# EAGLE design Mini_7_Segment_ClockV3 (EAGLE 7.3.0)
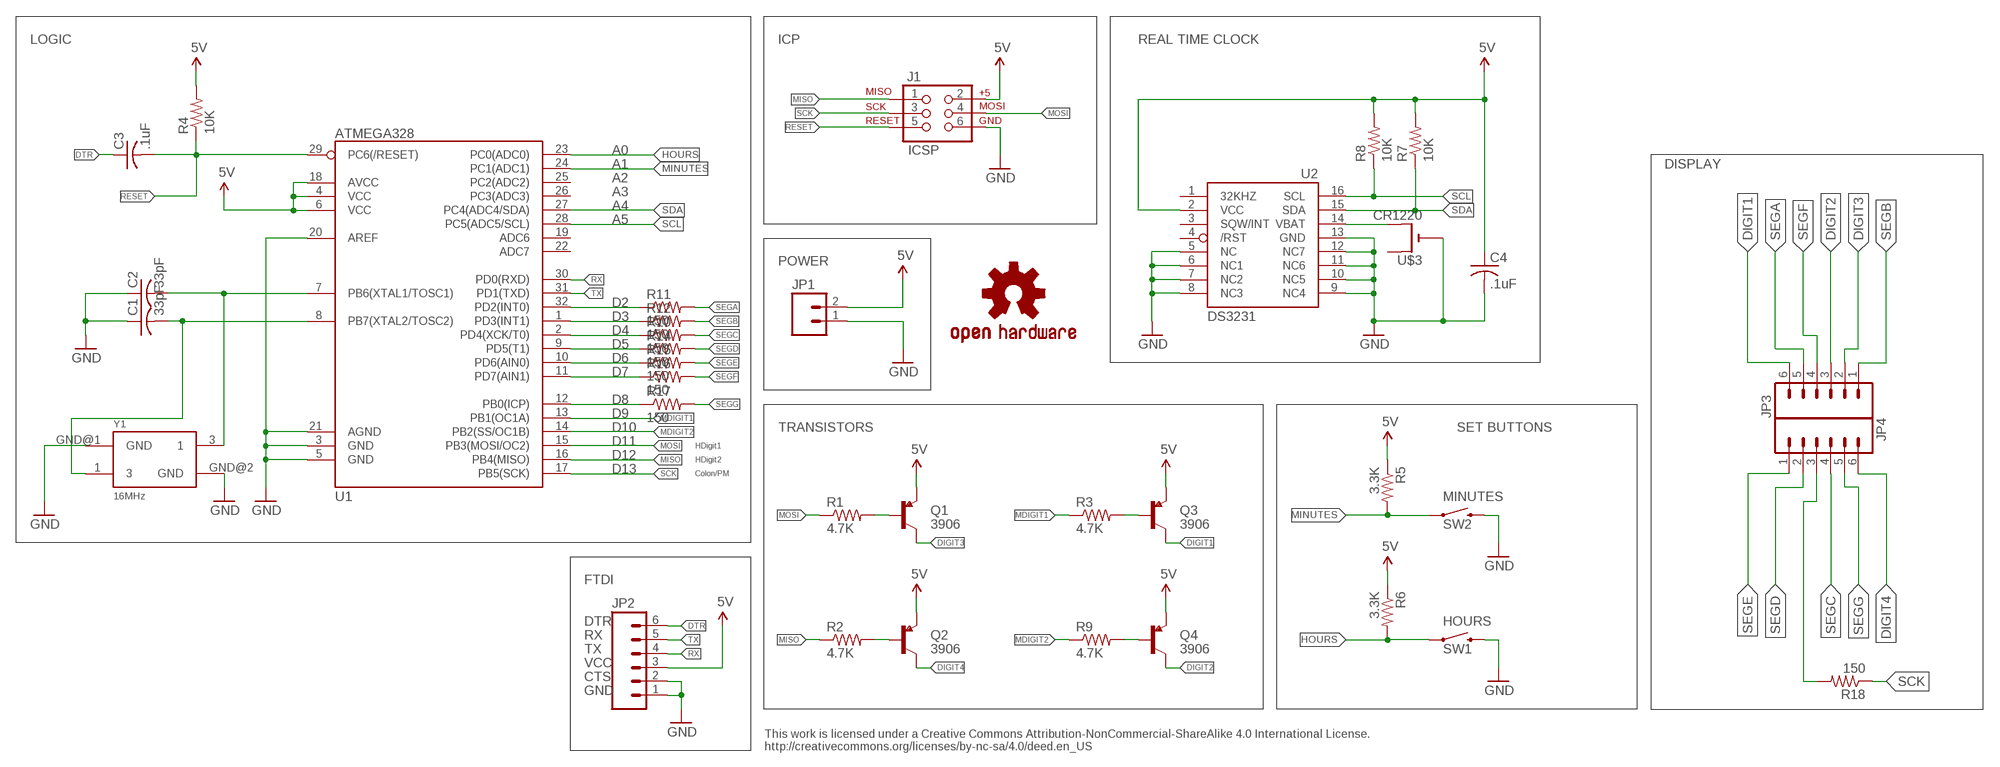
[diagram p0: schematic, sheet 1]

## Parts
C1  33pF  C-USC0805K  [C0805K]
C2  33pF  C-USC0805K  [C0805K]
C3  .1uF  C-USC0805K  [C0805K]
C4  .1uF  C-USC0805K  [C0805K]
HOURS  SW1  SWITCH-MOMENTARY-2PTH  [TACTILE-PTH]
J1  ICSP  AVR_SPI_PRG_6PTH  [2X3]
JP1  M02PTH  [1X02]
JP2  M06NO_SILK_FEMALE_PTH  [1X06_NO_SILK]
JP3  M06NO_SILK_FEMALE_PTH  [1X06_NO_SILK]
JP4  M06NO_SILK_FEMALE_PTH  [1X06_NO_SILK]
MINUTES  SW2  SWITCH-MOMENTARY-2PTH  [TACTILE-PTH]
Q1  3906  TRANSISTOR_PNPPMBT3906  [SOT23-3]
Q2  3906  TRANSISTOR_PNPPMBT3906  [SOT23-3]
Q3  3906  TRANSISTOR_PNPPMBT3906  [SOT23-3]
Q4  3906  TRANSISTOR_PNPPMBT3906  [SOT23-3]
R1  4.7K  R-US_R0805  [R0805]
R2  4.7K  R-US_R0805  [R0805]
R3  4.7K  R-US_R0805  [R0805]
R4  10K  R-US_R0805  [R0805]
R5  3.3K  R-US_R0805  [R0805]
R6  3.3K  R-US_R0805  [R0805]
R7  10K  R-US_R0805  [R0805]
R8  10K  R-US_R0805  [R0805]
R9  4.7K  R-US_R0805  [R0805]
R10  150  R-US_R0805  [R0805]
R11  150  R-US_R0805  [R0805]
R12  150  R-US_R0805  [R0805]
R14  150  R-US_R0805  [R0805]
R15  150  R-US_R0805  [R0805]
R16  150  R-US_R0805  [R0805]
R17  150  R-US_R0805  [R0805]
R18  150  R-US_R0805  [R0805]
U1  ATMEGA328  ATMEGA328_SMT  [TQFP32-08]
U2  DS3231  DS3231/SO  [SO16W]
U$3  CR1220  CR1220SMT  [CR1220-SMD]
U$7  OSHW-LOGOS  [OSHW-LOGO-S]
Y1  16MHz  OSCILLATOR5X3  [CRYSTAL-SMD-5X3]

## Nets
5V: C4.1 J1.2 JP1.2 JP2.3 Q1.2(E) Q2.2(E) Q3.2(E) Q4.2(E) R4.2 R5.1 R6.1 R7.2 R8.2 U1.4(VCC) U1.6(VCC) U1.18(AVCC) U2.2(VCC)
DIGIT1: JP3.6 Q3.3(C)
DIGIT2: JP3.3 Q4.3(C)
DIGIT3: JP3.2 Q1.3(C)
DIGIT4: JP4.6 Q2.3(C)
DTR: C3.1 JP2.6
GND: C1.1 C2.1 C4.2 HOURS.3 J1.6 JP1.1 JP2.1 JP2.2 MINUTES.3 U1.3(GND) U1.5(GND) U1.20(AREF) U1.21(AGND) U2.5(NC) U2.6(NC1) U2.7(NC2) U2.8(NC3) U2.9(NC4) U2.10(NC5) U2.11(NC6) U2.12(NC7) U2.13(GND) U$3.- Y1.GND@1(GND) Y1.GND@2(GND)
HOURS: HOURS.1 R6.2 U1.23(PC0(ADC0))
MDIGIT1: R3.1 U1.13(PB1(OC1A))
MDIGIT2: R9.1 U1.14(PB2(SS/OC1B))
MINUTES: MINUTES.1 R5.2 U1.24(PC1(ADC1))
MISO: J1.1 R2.1 U1.16(PB4(MISO))
MOSI: J1.4 R1.1 U1.15(PB3(MOSI/OC2))
N$1: R10.1 U1.2(PD4(XCK/T0))
N$2: JP4.3 R18.2
N$3: Q1.1(B) R1.2
N$4: R12.1 U1.1(PD3(INT1))
N$5: Q2.1(B) R2.2
N$6: Q3.1(B) R3.2
N$7: Q4.1(B) R9.2
N$8: C1.2 U1.8(PB7(XTAL2/TOSC2)) Y1.1
N$9: R16.1 U1.11(PD7(AIN1))
N$10: C2.2 U1.7(PB6(XTAL1/TOSC1)) Y1.3
N$11: R17.1 U1.12(PB0(ICP))
N$12: R14.1 U1.9(PD5(T1))
N$13: R11.1 U1.32(PD2(INT0))
N$14: R15.1 U1.10(PD6(AIN0))
N$15: U2.14(VBAT) U$3.+$2(+1)
RESET: C3.2 J1.5 R4.1 U1.29(PC6(/RESET))
RX: JP2.4 U1.30(PD0(RXD))
SCK: J1.3 R18.1 U1.17(PB5(SCK))
SCL: R8.1 U1.28(PC5(ADC5/SCL)) U2.16(SCL)
SDA: R7.1 U1.27(PC4(ADC4/SDA)) U2.15(SDA)
SEGA: JP3.5 R11.2
SEGB: JP3.1 R12.2
SEGC: JP4.4 R10.2
SEGD: JP4.2 R14.2
SEGE: JP4.1 R15.2
SEGF: JP3.4 R16.2
SEGG: JP4.5 R17.2
TX: JP2.5 U1.31(PD1(TXD))
Unconnected: U1.19(ADC6) U1.22(ADC7) U1.25(PC2(ADC2)) U1.26(PC3(ADC3)) U2.1(32KHZ) U2.3(SQW/INT) U2.4(/RST) U$3.+$1(+)

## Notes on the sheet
- LOGIC | ICP | REAL TIME CLOCK
- A0
- A1 | DISPLAY
- A2
- A3
- A4
- A5
- POWER
- D2
- D3
- D4
- D5
- D6
- D7
- D8
- D9
- D10 | TRANSISTORS | SET BUTTONS
- D11 | HDigit1
- D12 | HDigit2
- D13 | Colon/PM
- FTDI
- DTR
- RX
- TX
- VCC
- CTS
- GND
- This work is licensed under a Creative Commons Attribution-NonCommercial-ShareAlike 4.0 International License.
  http://creativecommons.org/licenses/by-nc-sa/4.0/deed.en_US

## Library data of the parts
C1-C4 = adafruit:C-US: CAPACITOR, American symbol
HOURS MINUTES = SparkFun:SWITCH-MOMENTARY-2
J1 = SparkFun:AVR_SPI_PRG_6: AVR ISP 6 Pin This is the reduced ISP connector for AVR programming. Common on Arduino. This footprint will take up less PCB space and can be used with a 10-pin to 6-pin adapter such as SKU: BOB-08508; OC_NEWARK: unknown
JP1 = SparkFun-Connectors:M02: Header 2
JP2-JP4 = SparkFun-Connectors:M06: Header 6 Standard 6-pin 0.1" header. Use with straight break away headers (SKU : PRT-00116), right angle break away headers (PRT-00553), swiss pins (PRT-00743), machine pins (PRT-00117), and female headers (PRT-00115). Molex polarized connector foot print use with SKU : PRT-08094 with associated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; PROD_ID: CONN-08437
Q1-Q4 = SparkFun-DiscreteSemi:TRANSISTOR_PNP: Generic PNP BJT Double check pinouts against datasheets- not all devices are the same! MMBT3906 - 40V 200mA SOT-23 (TRANS-08052) MMBT4403 - 40V 600mA SOT-23 (TRANS-09245); PROD_ID: TRANS-08052; VALUE: PMBT3906
R1-R12 R14-R18 = adafruit:R-US_: RESISTOR, American symbol
U1 = SparkFun-DigitalIC:ATMEGA328_SMT: 32-Pin Atmega328 part Commonly used on Arduino compatible boards Available in QFP and QFN packages TQFP is IC-09069 QFN is non-stock; PROD_ID: IC-09069; VALUE: ATMEGA328P
U2 = adafruit:DS3231
U$3 = adafruit:CR1220: CR1216/CR1220/CR1225 12mm 3V lithium coin cell Great for battery packup. Both SMT and THM holders. Note the THM package has the ground pads on both sides of the PCB so that the masks are the same - this reduces the cost
U$7 = SparkFun:OSHW-LOGO: Open Source Hardware Logo This logo indicates the piece of hardware it is found on incorporates a OSHW license and/or adheres to the definition of open source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
Y1 = SparkFun-FreqCtrl:OSCILLATOR: Generic 5x3 and 7x5 oscillators

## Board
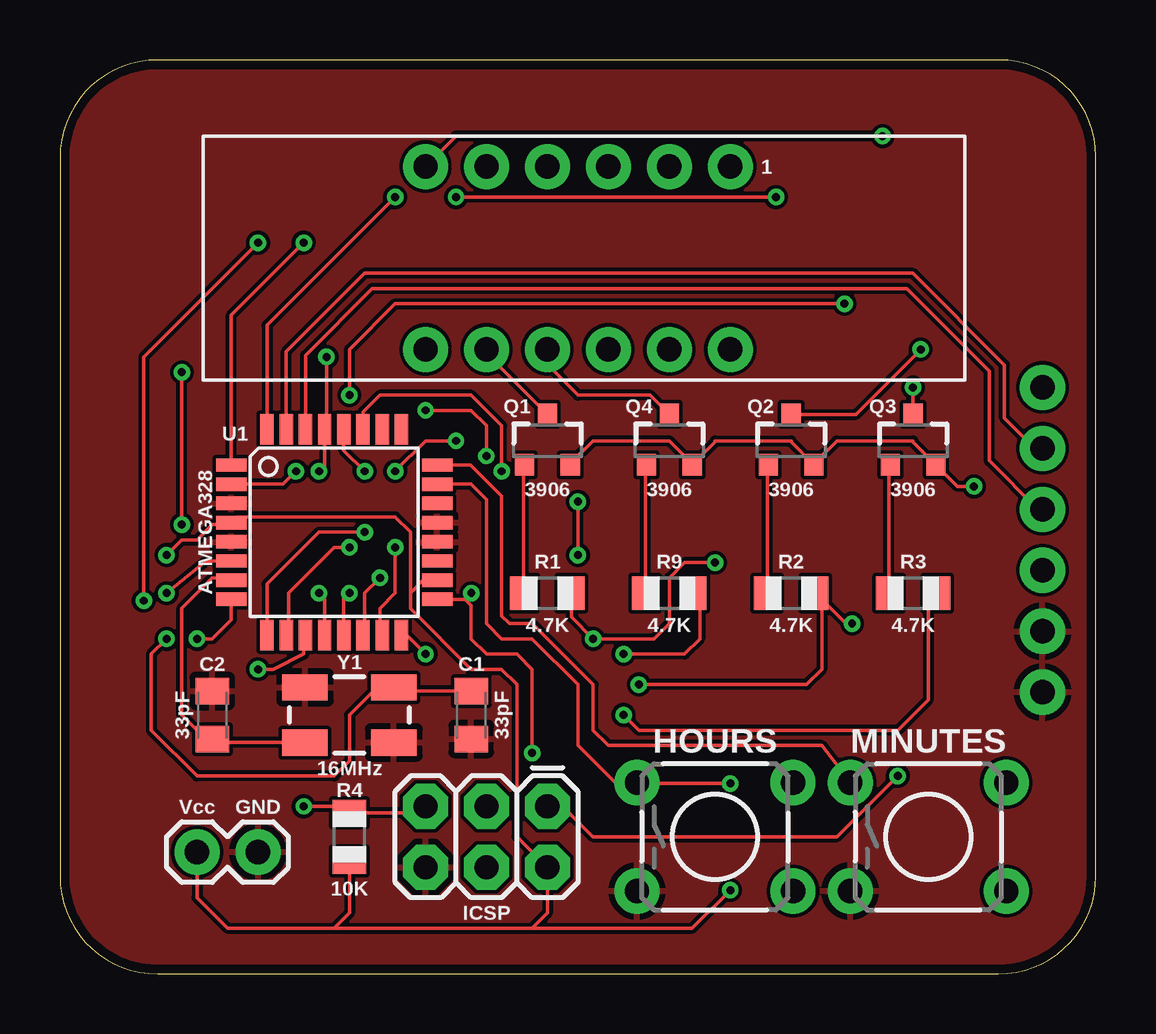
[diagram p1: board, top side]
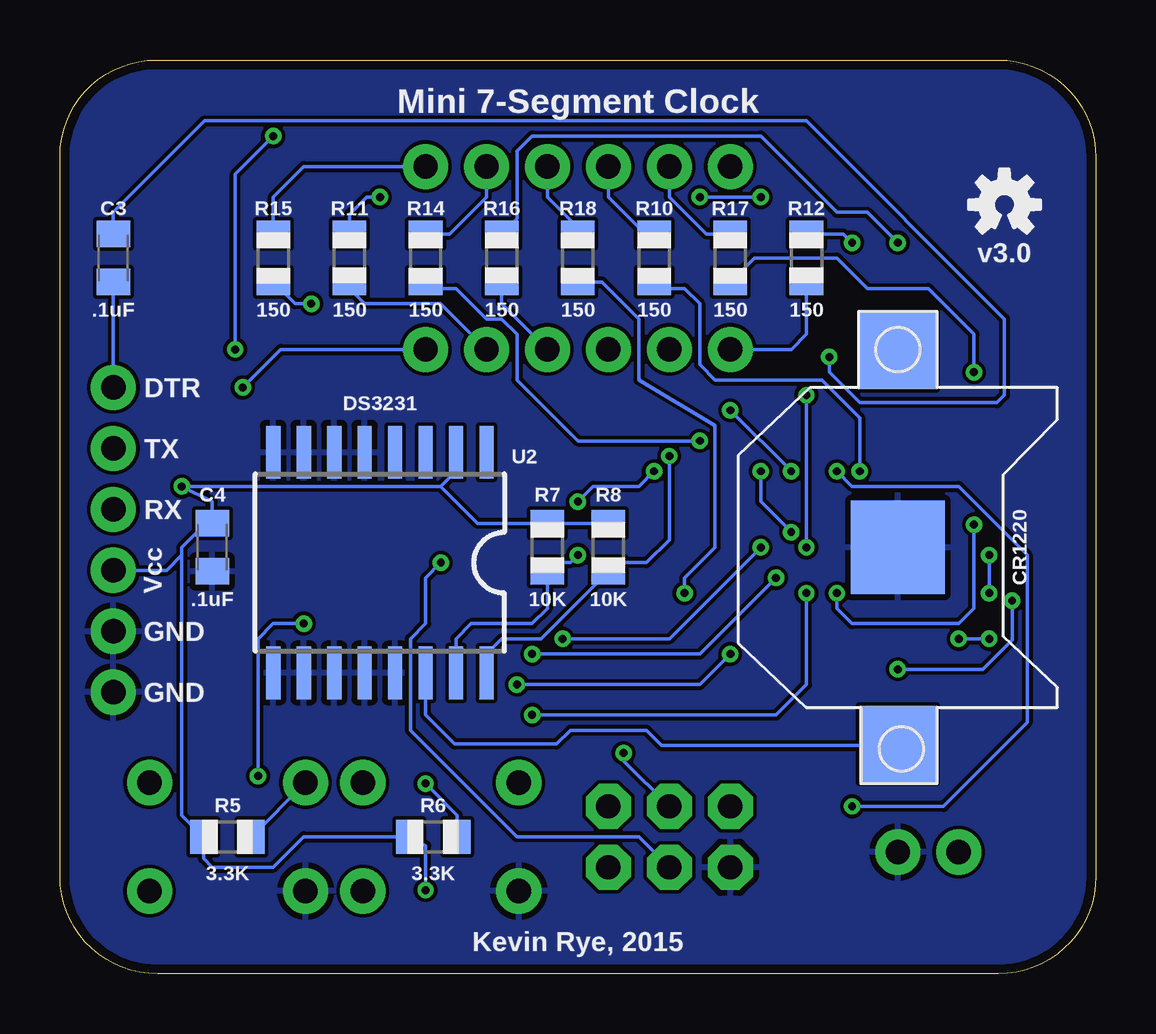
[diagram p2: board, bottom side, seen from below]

Size 43.18 x 38.1 mm. Coordinates in mm from the lower left corner, seen from the top.
Outline: 0,34.03 0,4.07 arc90 4.07,0 39.11,0 arc90 43.18,4.07 43.18,34.08 arc90 39.16,38.1 4.07,38.1 arc90 0,34.03
Copper layers (1*16): Top 0.0356mm / dielectric 1.5011mm / Bottom 0.0356mm
Design rules "LaenPCBOrder": minimum track width 6mil, minimum drill 13mil, track to track 6mil, track to pad 6mil, pad to pad 6mil, via to via 6mil, smd to smd 6mil, copper to edge 15mil, drill to drill 6mil, minimum pad ring 7mil, minimum via ring 7mil, stop-mask expansion 3mil, vias tented up to drill 0mil, thermal gap 10mil

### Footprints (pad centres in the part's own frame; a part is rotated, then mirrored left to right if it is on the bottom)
C0805K = smd 1.1 x 1.4: 1 -1,0; 2 1,0
TACTILE-PTH = drill 1.016 pad 1.88: 1 -3.251,2.261; 2 3.251,2.261; 3 -3.251,-2.261; 4 3.251,-2.261
2X3 = drill 1.016 pad 1.88 octagon: 1 0,0; 2 0,2.54; 3 2.54,0; 4 2.54,2.54; 5 5.08,0; 6 5.08,2.54
1X02 = drill 1.016 pad 1.88: 1 0,0; 2 2.54,0
1X06_NO_SILK = drill 1.016 pad 1.88: 1 0,0; 2 2.54,0; 3 5.08,0; 4 7.62,0; 5 10.16,0; 6 12.7,0
SOT23-3 = smd 0.8 x 0.9: 1 -0.95,-1; 2 0.95,-1; 3 0,1.1
R0805 = smd 1.1 x 1.4: 1 -1,0; 2 1,0
TQFP32-08 = smd 1.27 x 0.559: 1 -4.293,2.8; 2 -4.293,2; 3 -4.293,1.2; 4 -4.293,0.4; 5 -4.293,-0.4; 6 -4.293,-1.2; 7 -4.293,-2; 8 -4.293,-2.8; 17 4.293,-2.8; 18 4.293,-2; 19 4.293,-1.2; 20 4.293,-0.4; 21 4.293,0.4; 22 4.293,1.2; 23 4.293,2; 24 4.293,2.8 | smd 0.559 x 1.27: 9 -2.8,-4.293; 10 -2,-4.293; 11 -1.2,-4.293; 12 -0.4,-4.293; 13 0.4,-4.293; 14 1.2,-4.293; 15 2,-4.293; 16 2.8,-4.293; 25 2.8,4.293; 26 2,4.293; 27 1.2,4.293; 28 0.4,4.293; 29 -0.4,4.293; 30 -1.2,4.293; 31 -2,4.293; 32 -2.8,4.293
SO16W = smd 0.6 x 2.2: 1 -4.445,-4.6; 2 -3.175,-4.6; 3 -1.905,-4.6; 4 -0.635,-4.6; 5 0.635,-4.6; 6 1.905,-4.6; 7 3.175,-4.6; 8 4.445,-4.6; 9 4.445,4.6; 10 3.175,4.6; 11 1.905,4.6; 12 0.635,4.6; 13 -0.635,4.6; 14 -1.905,4.6; 15 -3.175,4.6; 16 -4.445,4.6
CR1220-SMD = smd 3.2 x 3.2: +$1 -8.2,0; +$2 8.2,0 | smd 3.9 x 3.9: - 0,0
CRYSTAL-SMD-5X3 = smd 1.9 x 1.1: 1 -1.85,-1.15; 3 1.85,1.15; GND@1 -1.85,1.15; GND@2 1.85,-1.15

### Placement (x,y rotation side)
C1  17.14,10.79 90 top
C2  6.35,10.79 270 top
C3  40.96,29.85 90 bottom
C4  36.83,17.78 270 bottom
HOURS  27.3,5.71 0 top
J1  20.32,6.98 180 top
JP1  8.26,5.08 180 top
JP2  40.96,11.75 90 bottom
JP3  15.24,26.04 0 top
JP4  27.94,33.66 180 top
MINUTES  36.2,5.71 0 top
Q1  20.32,22.23 0 top
Q2  30.48,22.23 0 top
Q3  35.56,22.23 0 top
Q4  25.4,22.23 0 top
R1  20.32,15.88 180 top
R2  30.48,15.88 180 top
R3  35.56,15.88 180 top
R4  12.06,5.71 270 top
R5  36.2,5.71 0 bottom
R6  27.62,5.71 0 bottom
R7  22.86,17.78 90 bottom
R8  20.32,17.78 90 bottom
R9  25.4,15.88 180 top
R10  18.41,29.85 90 bottom
R11  31.11,29.85 270 bottom
R12  12.06,29.85 270 bottom
R14  27.94,29.85 90 bottom
R15  34.29,29.85 90 bottom
R16  24.77,29.85 270 bottom
R17  15.24,29.85 90 bottom
R18  21.59,29.85 90 bottom
U1  11.43,18.42 0 top
U2  29.84,17.15 180 bottom
U$3  8.26,17.78 270 bottom
U$7  3.81,32.07 0 bottom
Y1  12.06,10.79 180 top

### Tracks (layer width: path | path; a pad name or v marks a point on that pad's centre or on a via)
5V  (via drill 0.33 pad 0.69)
  Top 0.152: JP1.2 5.71,3.17 6.98,1.91 11.43,1.91 | 11.43,1.91 19.68,1.91 | 19.68,1.91 26.35,1.91 v27.94,3.49 | 19.68,1.91 20.32,2.54 J1.2 19.05,5.71 19.05,12.06 18.41,12.7 17.14,12.7 14.61,15.24 14.61,15.88 | R4.2 12.06,2.54 11.43,1.91 | Q1.2 21.27,21.27 22.22,22.23 25.4,22.23 26.35,21.28 | 26.35,21.28 Q4.2 27.3,22.18 27.3,22.23 30.48,22.23 30.48,22.18 Q2.2 31.43,21.27 32.38,22.23 35.56,22.23 35.56,22.18 Q3.2 37.42,20.32 v38.1,20.32 | 26.35,21.28 26.36,21.28 | U1.6 6.1,17.21 v4.45,15.88 | U1.18 15.14,16.41 14.61,15.88 | 14.61,15.88 14.61,18.42 13.97,19.05 7.37,19.05 U1.4 7.05,18.73 6.35,18.73 5.71,18.1 5.08,18.1 v4.45,17.46
  Bottom 0.152: v27.94,3.49 27.94,5.35 R6.1 33.02,5.71 34.29,4.45 36.83,4.45 37.2,4.81 R5.1 38.1,6.62 38.1,17.46 | 38.1,17.46 38.1,17.78 37.1,18.78 C4.1 36.83,19.69 v38.1,20.32 27.3,20.32 | U2.2 26.67,20.96 27.3,20.32 | 27.3,20.32 25.77,18.78 R7.2 R8.2 | v4.45,15.88 v4.45,17.46 | JP2.3 38.74,16.83 38.1,17.46
DIGIT1  (via drill 0.33 pad 0.69)
  Top 0.152: Q3.3 v35.56,24.45
  Bottom 0.152: v35.56,24.45 33.97,26.04 JP3.6
DIGIT2
  Top 0.152: Q4.3 24.59,24.13 21.59,24.13 20.32,25.4 JP3.3
DIGIT3
  Top 0.152: Q1.3 17.78,25.87 JP3.2
DIGIT4  (via drill 0.33 pad 0.69)
  Top 0.152: Q2.3 33.17,23.33 v35.88,26.04 | v34.29,34.92 16.51,34.92 JP4.6
  Bottom 0.152: v35.88,26.04 35.88,33.34 v34.29,34.92
DTR
  Bottom 0.152: C3.1 JP2.6
GND
  pour Bottom: -0.64,38.73 43.82,39.05 43.82,-0.64 -0.64,-0.64
  pour Top: -0.32,38.42 43.5,38.42 43.5,-0.32 -0.32,-0.32
HOURS  (via drill 0.33 pad 0.69)
  Top 0.152: U1.23 17.14,20.42 17.78,19.77 17.78,14.61 18.41,13.97 19.68,13.97 21.59,12.06 21.59,9.53 23.14,7.98 HOURS.1 24.09,7.94 v27.94,7.94
  Bottom 0.152: R6.2 26.62,6.62 v27.94,7.94
MDIGIT1  (via drill 0.33 pad 0.69)
  Top 0.152: R3.1 36.2,15.88 36.2,11.43 34.93,10.16 24.13,10.16 v23.5,10.79 | v12.06,15.88 11.83,15.64 U1.13
  Bottom 0.152: v23.5,10.79 13.33,10.79 12.06,12.06 v12.06,15.88
MDIGIT2  (via drill 0.33 pad 0.69)
  Top 0.152: R9.1 26.67,15.61 26.67,13.97 26.04,13.33 v23.5,13.33 | v13.33,16.51 12.7,15.88 12.7,14.12 U1.14
  Bottom 0.152: v23.5,13.33 16.51,13.33 v13.33,16.51
MINUTES
  Top 0.152: U1.24 17.12,21.21 18.41,19.92 18.41,14.92 18.73,14.61 19.68,14.61 22.22,12.06 22.22,10.16 22.86,9.53 31.75,9.53 MINUTES.1
  Bottom 0.152: MINUTES.1 R5.2
MISO  (via drill 0.33 pad 0.69)
  Top 0.152: v24.13,12.06 31.11,12.06 31.75,12.7 31.75,15.61 R2.1 32.75,14.61 v33.02,14.61 | v15.24,13.33 14.45,14.12 U1.16 | J1.1 20.95,6.98 22.22,5.71 32.38,5.71 v34.93,8.26
  Bottom 0.152: v24.13,12.06 16.51,12.06 v15.24,13.33 | v34.93,8.26 34.93,13.97 34.29,14.61 v33.02,14.61
MOSI  (via drill 0.33 pad 0.69)
  Top 0.152: R1.1 21.32,14.88 v22.22,13.97 24.77,13.97 25.4,14.61 25.4,16.51 26.04,17.15 v27.3,17.15 | v13.97,17.78 13.97,15.88 13.33,15.24 13.33,14.22 U1.15
  Bottom 0.152: v22.22,13.97 17.78,13.97 v13.97,17.78 | J1.4 19.05,5.71 24.13,5.71 28.57,10.16 28.57,13.97 27.94,14.61 27.94,16.51 v27.3,17.15
N$1  (via drill 0.33 pad 0.69)
  Top 0.152: v9.84,20.96 9.3,20.42 U1.2
  Bottom 0.152: R10.1 18.14,28.58 17.14,28.58 16.51,27.94 16.51,25.4 15.88,24.77 11.43,24.77 9.84,23.18 v9.84,20.96
N$2
  Bottom 0.152: R18.2 21.59,31.12 22.86,32.38 JP4.3
N$3
  Top 0.152: R1.2 19.32,21.18 Q1.1
N$4  (via drill 0.33 pad 0.69)
  Top 0.152: U1.1 7.14,27.46 v10.16,30.48
  Bottom 0.152: v10.16,30.48 10.53,30.85 R12.1
N$5
  Top 0.152: R2.2 29.48,21.18 Q2.1
N$6
  Top 0.152: R3.2 34.56,21.18 Q3.1
N$7
  Top 0.152: R9.2 24.4,21.18 Q4.1
N$8  (via drill 0.33 pad 0.69)
  Top 0.152: C1.2 14.06,11.79 Y1.1 13.21,11.95 12.06,10.79 12.06,8.89 11.43,8.26 5.71,8.26 3.81,10.16 3.81,13.33 v4.45,13.97 | U1.8 7.14,14.76 6.35,13.97 v5.71,13.97
  Bottom 0.152: v5.71,13.97 v4.45,13.97
N$9  (via drill 0.33 pad 0.69)
  Top 0.152: v8.26,30.48 3.49,25.72 v3.49,15.56 | v8.26,12.7 8.89,12.7 10.16,13.33 10.16,14.05 U1.11
  Bottom 0.152: R16.1 24.13,31.48 24.13,34.29 23.5,34.92 13.97,34.92 10.79,31.75 9.53,31.75 v8.26,30.48 | v3.49,15.56 3.49,13.92 4.71,12.7 v8.26,12.7
N$10
  Top 0.152: Y1.3 6.5,9.64 C2.2 6.08,9.79 5.08,10.79 5.08,15.24 6.35,16.51 7.04,16.51 U1.7
N$11  (via drill 0.33 pad 0.69)
  Top 0.152: v10.79,15.88 11.03,15.64 U1.12 | v5.08,18.73 v5.08,25.08
  Bottom 0.152: R17.1 14.24,29.85 10.79,29.85 9.53,28.58 6.98,28.58 5.08,26.67 v5.08,25.08 | v10.79,15.88 10.79,15.24 10.16,14.61 5.71,14.61 5.08,15.24 v5.08,18.73
N$12  (via drill 0.33 pad 0.69)
  Top 0.152: v16.51,22.23 15.24,22.23 v13.97,20.96 | U1.9 8.63,16.25 10.79,18.42 v12.7,18.42
  Bottom 0.152: R14.1 27.67,28.58 26.67,28.58 25.4,27.31 24.77,27.31 24.13,26.67 24.13,24.77 21.59,22.23 v16.51,22.23 | v12.7,18.42 13.97,19.69 v13.97,20.96
N$13  (via drill 0.33 pad 0.69)
  Top 0.152: v29.84,32.38 v16.51,32.38 | v13.97,32.38 8.63,27.05 U1.32
  Bottom 0.152: R11.1 31.11,31.68 30.41,32.38 v29.84,32.38 | v16.51,32.38 v13.97,32.38
N$14  (via drill 0.33 pad 0.69)
  Top 0.152: U1.10 9.53,14.22 9.53,15.88 11.43,17.78 v12.06,17.78 | v12.06,24.13 12.06,26.04 13.97,27.94 v32.7,27.94
  Bottom 0.152: v12.06,17.78 v12.06,24.13 | v32.7,27.94 33.39,27.94 R15.1
N$15
  Bottom 0.152: U2.14 27.94,10.79 26.72,9.58 22.49,9.58 21.91,10.16 18.73,10.16 18.1,9.53 8.31,9.53 U$3.+$2
RESET  (via drill 0.33 pad 0.69)
  Top 0.152: J1.5 14.97,6.71 R4.1 11.79,6.98 v10.16,6.98 | v10.79,20.96 11.03,21.19 U1.29 11.11,22.79 v11.11,25.72
  Bottom 0.152: v10.79,20.96 10.16,20.32 5.71,20.32 2.86,17.46 2.86,10.48 6.35,6.98 v10.16,6.98 | 40.96,31.12 C3.2 40.96,31.75 37.15,35.56 12.06,35.56 3.81,27.31 3.81,24.13 4.13,23.81 9.84,23.81 11.11,25.08 v11.11,25.72
RX
  Top 0.152: U1.30 10.23,25.79 13.02,28.58 35.3,28.58 38.74,25.14 38.74,21.4 40.77,19.37 JP2.4
SCK  (via drill 0.33 pad 0.69)
  Top 0.152: v17.14,15.88 16.89,15.62 | 16.89,15.62 U1.17 | 16.89,15.62 17.14,15.36 17.14,13.97 17.78,13.33 19.05,13.33 19.68,12.7 v19.68,9.21
  Bottom 0.152: R18.1 20.59,28.85 19.05,27.31 19.05,24.77 15.88,22.86 15.88,17.78 17.14,16.51 v17.14,15.88 | v19.68,9.21 19.68,8.89 J1.3
SCL  (via drill 0.33 pad 0.69)
  Top 0.152: v17.78,21.59 17.78,22.86 17.14,23.5 v15.24,23.5 | v12.7,20.96 11.83,21.83 U1.28
  Bottom 0.152: U2.16 25.4,13.33 24.77,13.97 23.13,13.97 R8.1 19.95,17.15 18.73,17.15 17.78,18.1 v17.78,21.59 | v15.24,23.5 v12.7,20.96
SDA  (via drill 0.33 pad 0.69)
  Top 0.152: v18.41,20.96 18.41,22.86 17.14,24.13 13.33,24.13 12.63,23.43 U1.27 | v21.59,17.46 v21.59,19.69
  Bottom 0.152: U2.15 26.67,13.97 26.04,14.61 23.5,14.61 22.86,15.24 R7.1 22.59,16.78 22.22,17.15 21.91,17.15 v21.59,17.46 | v18.41,20.96 19.05,20.32 20.95,20.32 v21.59,19.69
SEGA
  Bottom 0.152: JP3.5 27.3,27.94 30.48,27.94 31.11,28.58 R11.2
SEGB
  Bottom 0.152: JP3.1 12.7,26.04 12.06,26.67 R12.2
SEGC
  Bottom 0.152: R10.2 18.78,30.85 20.32,32.38 JP4.4
SEGD
  Bottom 0.152: R14.2 26.94,30.85 25.4,32.38 JP4.2
SEGE
  Bottom 0.152: R15.2 34.29,32.38 33.02,33.66 JP4.1
SEGF
  Bottom 0.152: JP3.4 24.77,27.94 R16.2
SEGG
  Bottom 0.152: R17.2 16.24,30.85 17.78,32.38 JP4.5
TX
  Top 0.152: U1.31 9.43,25.94 12.7,29.21 35.55,29.21 39.37,25.39 39.37,23.18 40.64,21.91 JP2.5

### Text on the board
Unrouted: This work is licensed under a Creative Commons Attribution-NonCommercial-ShareAlike 4.0 International License. / http://creativecommons.org/licenses/by-nc-sa/4.0/deed.en_US
tPlace: 1 | Vcc | GND
bPlace: Mini 7-Segment Clock | v3.0 | DTR | TX | RX | Vcc | GND | GND | Kevin Rye, 2015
